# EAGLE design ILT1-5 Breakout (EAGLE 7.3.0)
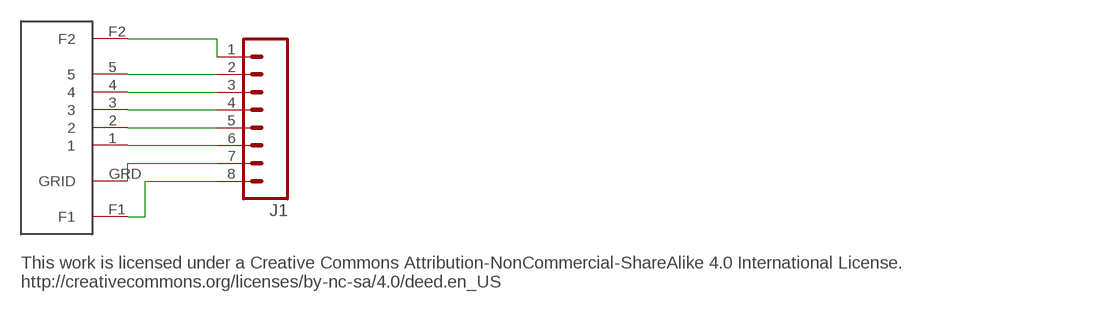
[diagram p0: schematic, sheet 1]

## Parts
J1  M08  [1X08_ROUND]
U$1  ILT1-5L  [ILT1-5L]

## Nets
N$1: J1.1 U$1.F2
N$2: J1.2 U$1.5
N$3: J1.3 U$1.4
N$4: J1.4 U$1.3
N$5: J1.5 U$1.2
N$6: J1.6 U$1.1
N$7: J1.7 U$1.GRD(GRID)
N$8: J1.8 U$1.F1

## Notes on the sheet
- This work is licensed under a Creative Commons Attribution-NonCommercial-ShareAlike 4.0 International License.
  http://creativecommons.org/licenses/by-nc-sa/4.0/deed.en_US

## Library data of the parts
J1 = SparkFun-Connectors:M08: Header 8 Standard 8-pin 0.1" header. Use with straight break away headers (SKU : PRT-00116), right angle break away headers (PRT-00553), swiss pins (PRT-00743), machine pins (PRT-00117), and female headers (PRT-00115).; PROD_ID: CONN-08437
U$1 = ILT1-5 L:ILT1-5L

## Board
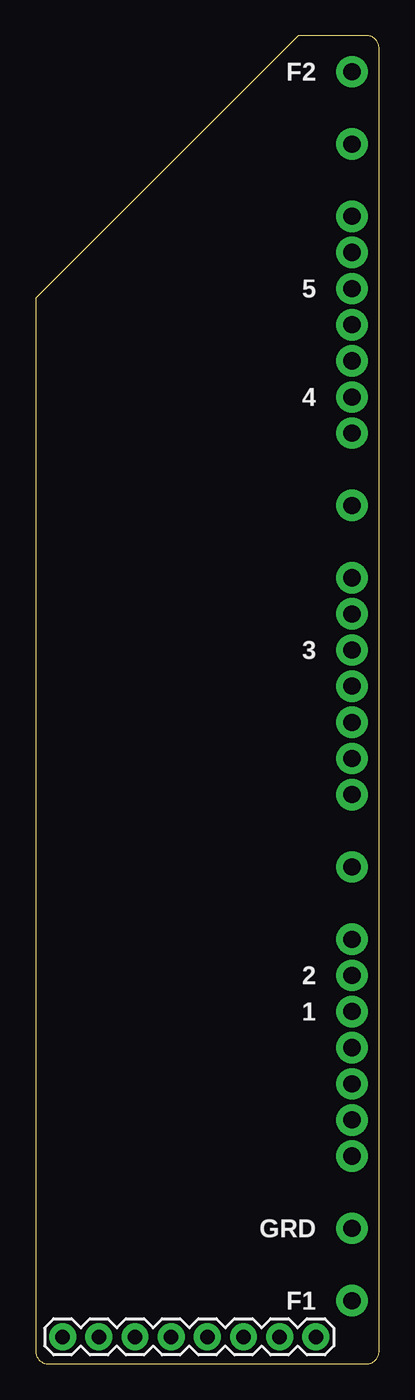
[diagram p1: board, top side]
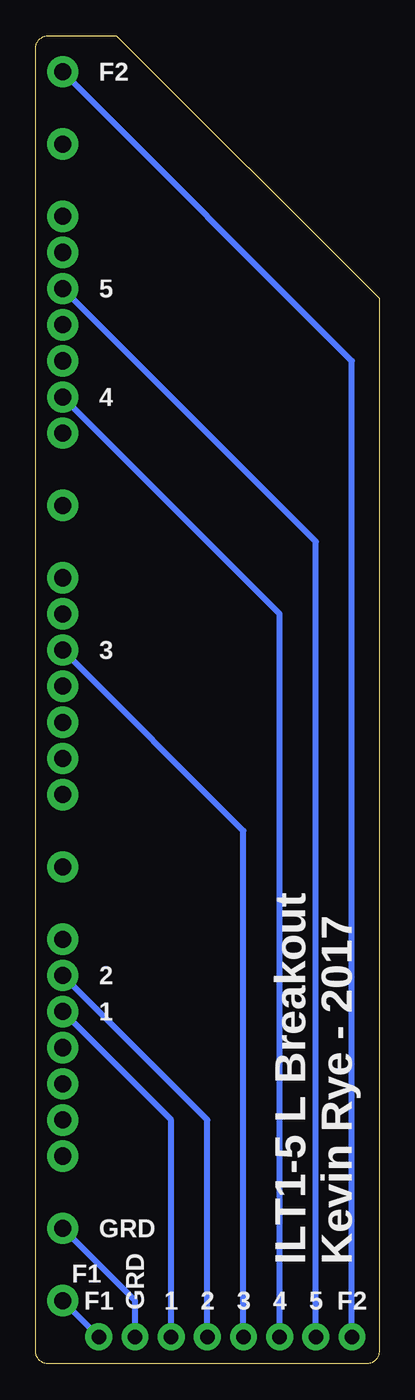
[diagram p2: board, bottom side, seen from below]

Size 24.13 x 93.34 mm. Coordinates in mm from the lower left corner, seen from the top.
Outline: 23.23,93.34 18.46,93.34 0,74.89 0,0.9 arc90 0.9,0 23.23,0 arc90 24.13,0.9 24.13,92.45 arc90 23.23,93.34
Copper layers (1*16): Top 0.0356mm / dielectric 1.5011mm / Bottom 0.0356mm
Design rules "oshpark-2layer": minimum track width 6mil, minimum drill 13mil, track to track 6mil, track to pad 6mil, pad to pad 6mil, via to via 6mil, smd to smd 6mil, copper to edge 15mil, drill to drill 6mil, minimum pad ring 7mil, minimum via ring 7mil, stop-mask expansion 2.5mil, vias tented up to drill 0mil, thermal gap 10mil

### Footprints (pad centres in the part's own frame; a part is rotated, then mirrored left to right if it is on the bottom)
1X08_ROUND = drill 1.016 pad 1.88: 1 0,0; 2 2.54,0; 3 5.08,0; 4 7.62,0; 5 10.16,0; 6 12.7,0; 7 15.24,0; 8 17.78,0
ILT1-5L = drill 1.2 pad 2.2: 1 0,20.32; 2 0,22.86; 3 0,45.72; 4 0,63.5; 5 0,71.12; F1 0,0; F2 0,86.36; GRD 0,5.08; P$5 0,12.7; P$6 0,10.16; P$7 0,15.24; P$8 0,17.78; P$11 0,25.4; P$13 0,30.48; P$15 0,35.56; P$16 0,38.1; P$17 0,40.64; P$18 0,43.18; P$20 0,48.26; P$21 0,50.8; P$23 0,55.88; P$25 0,60.96; P$27 0,66.04; P$28 0,68.58; P$30 0,73.66; P$31 0,76.2; P$33 0,81.28

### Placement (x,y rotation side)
J1  1.91,1.91 0 top
U$1  22.22,4.45 0 top

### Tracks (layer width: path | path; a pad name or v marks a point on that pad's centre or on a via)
N$1
  Bottom 0.406: J1.1 1.91,70.48 U$1.F2
N$2
  Bottom 0.406: J1.2 4.45,57.79 U$1.5
N$3
  Bottom 0.406: J1.3 6.99,52.71 U$1.4
N$4
  Bottom 0.406: J1.4 9.53,37.47 U$1.3
N$5
  Bottom 0.406: J1.5 12.06,17.14 U$1.2
N$6
  Bottom 0.406: J1.6 14.61,17.14 U$1.1
N$7
  Bottom 0.406: J1.7 17.14,4.45 U$1.GRD
N$8
  Bottom 0.406: J1.8 U$1.F1

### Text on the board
Unrouted: This work is licensed under a Creative Commons Attribution-NonCommercial-ShareAlike 4.0 International License. / http://creativecommons.org/licenses/by-nc-sa/4.0/deed.en_US
bNames: F2 | 5 | 4 | 3 | 2 | 1 | GRD | ILT1-5 L Breakout / Kevin Rye - 2017 | F1 | F2 | 5 | 4 | 3 | 2 | 1 | GRD | F1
